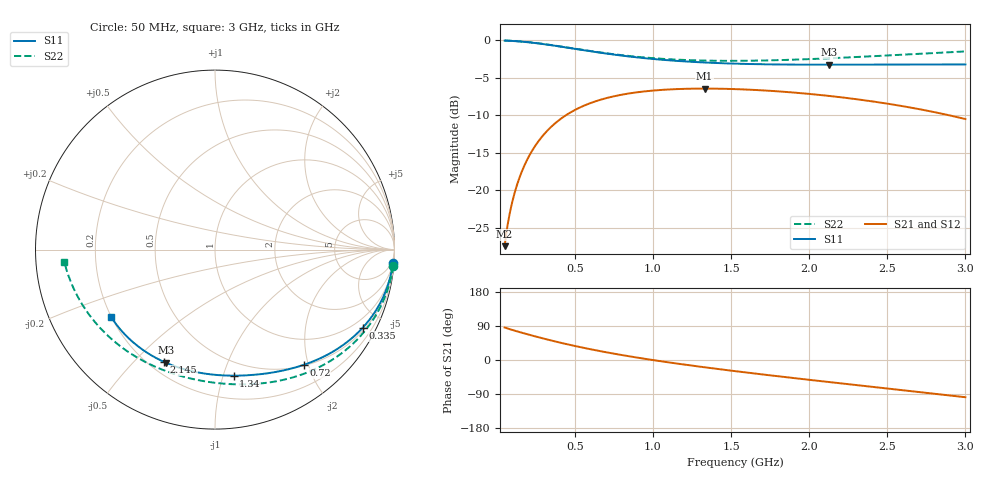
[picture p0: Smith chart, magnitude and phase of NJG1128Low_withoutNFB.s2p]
! NJG1128 Low Gain mode S-parameter
# hz S ma R 50	S	ma	R	50
! 2 Port Network Data from SP1.SP block	Port	Network	Data	from	SP1.SP	block
! freq  magS11  angS11  magS21  angS21  magS12  angS12  magS22  angS22  magS11	angS11	magS21	angS21	magS12	angS12	magS22	angS22
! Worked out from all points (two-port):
!   591 points, 50 MHz to 3 GHz, reference 50 ohm
!   highest |S21| = -6.44 dB at 1.33 GHz (marker M1); lowest = -27.4 dB at 50 MHz (marker M2)
!   |S21| within 3 dB of the highest: 486.6 MHz to 2.769 GHz (2.283 GHz wide, 140 % of centre)
!   lowest |S11| = -3.3 dB at 2.125 GHz (marker M3), VSWR 5.39, Z = 13.1 - j31.2 ohm
!   |S11| at or under -10 dB: nowhere
!   |S22| runs from -2.7 to 0.0 dB; largest |S21 - S12| = 1.6e-06
!   S11 on the Smith chart (normalised r, x): 50 MHz: 2, -26; 335 MHz: 0.60, -3.94; 720 MHz: 0.51, -1.92; 1.34 GHz: 0.38, -1.08; 2.145 GHz: 0.26, -0.61; 3 GHz: 0.20, -0.28
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5e7  0.9937 -4.4  0.0426 85.7  0.0426 85.7  0.9964 -5.3
8e7  0.9909 -7.0  0.06799 81.7  0.06799 81.7  0.9936 -8.4
1e8  0.9885 -8.8  0.08472 79.2  0.08472 79.2  0.9912 -10.5
1.25e8  0.9848 -10.9  0.1053 76.2  0.1053 76.2  0.9874 -13.1
1.55e8  0.9794 -13.5  0.1295 72.6  0.1295 72.6  0.982 -16.1
2.35e8  0.9606 -20.1  0.1904 63.5  0.1904 63.5  0.9631 -24.1
3.35e8  0.9309 -27.9  0.2573 52.8  0.2573 52.9  0.9332 -33.5
4.35e8  0.8979 -35.1  0.313 43.0  0.313 43.0  0.9001 -42.3
5.45e8  0.8616 -42.3  0.3618 33.0  0.3618 33.0  0.8641 -51.1
7.2e8  0.81 -52.5  0.4165 18.9  0.4165 18.9  0.814 -63.8
8.75e8  0.7734 -60.5  0.4469 7.9  0.4469 7.9  0.7799 -73.7
1.035e9  0.7445 -68.2  0.4655 -2.3  0.4655 -2.3  0.755 -83.2
1.33e9  0.7107 -81.2  0.4766 -19.2  0.4766 -19.2  0.7319 -99.0
1.34e9  0.7099 -81.6  0.4766 -19.7  0.4766 -19.7  0.7316 -99.5
1.525e9  0.6983 -89.4  0.4728 -29.4  0.4728 -29.4  0.7291 -108.8
1.775e9  0.6901 -99.6  0.4588 -41.7  0.4588 -41.7  0.7356 -120.8
2.02e9  0.6873 -109.4  0.4373 -53.2  0.4373 -53.2  0.75 -132.1
2.125e9  0.6871 -113.5  0.4262 -58.1  0.4262 -58.1  0.7579 -136.9
2.145e9  0.6871 -114.3  0.4239 -59.0  0.4239 -59.0  0.7595 -137.8
2.51e9  0.6886 -128.5  0.3769 -75.7  0.3769 -75.7  0.7925 -154.1
2.765e9  0.6897 -138.3  0.3381 -87.3  0.3381 -87.3  0.8182 -165.2
3e9  0.6898 -147.1  0.2987 -98.2  0.2987 -98.2  0.8423 -175.4
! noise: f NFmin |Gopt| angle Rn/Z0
5e+07  0.4555  0.9061  7.298  1.087
3.75e+08  0.6885  0.2152  87.47  0.09236
7.05e+08  1.067  0.3286  155.3  0.07436
1.03e+09  1.392  0.4266  169.5  0.07116
1.36e+09  1.696  0.4801  176.3  0.07252
1.685e+09  2.008  0.5113  -179.3  0.07733
2.015e+09  2.377  0.5324  -176  0.08605
2.34e+09  2.84  0.5476  -173.3  0.09989
2.67e+09  3.476  0.5598  -171.1  0.1228
3e+09  4.381  0.5699  -169.2  0.1628
